TYPE STR_NDO :
STRUCT
//	Heartbeat	,
	(*
	TUBRO_PUMO_POWER_ON	,
	PENDULUM_VALVE_POWER_ON	,
	LID_HEATER_POWER_ON	,
	CHAMBER_POWER_ON	,
	IGS_HEATER_POWER_ON	,
	TAPE_HEATER_POWER_ON	,
	FORLINE_HEATER_POWER_ON	,
	GATE_VALVE_HEATER_POWER_ON	,
	EV3_POWER_ON	,
	EV4_POWER_ON	,
	EV1_POWER_ON	,
	EV2_POWER_ON	,
	DRY_PUMP_RUN	,
	*)
	DRY_PUMP_RUN	,
	AV101	,
	AV102	,
	AV103	,
	AV104	,
	AV105	,
	AV106	,
	AV107	,
	AV108	,
	AV109	,	//pin middle
	AV110	,	//pin up
	GV101C	,	//门阀打开
	GV101O	,	//门阀关闭
	AV201	,
	AV202	,
	AC101	,
	AC102	,
	AC103	,
	AC104	,
	AC105	,
	AC106	,
	AV1		,
	AV2		,
	AV3		,
	AV4		,
	AV6		,
	AV7		,
	AV9		,
	AV10	,
	AV11	,
	AV12	,
	AV13	,
	AV14	,
	AV16	,
	AV17	,
	AV19	,
	AV20	,
	AV22	,
	AV23	,
	AV25	,
	AV26	,
	AV27	,
	AV5		,
	AV8		,
	AV15	,
	AV18	,
	AV21	,
	AV24	,
	MaualEndStep,
	GV_Open_Enable,
	GV_Close_Enable,
	TM_Robot_Extend_Enable	:BOOL;

END_STRUCT
END_TYPE
